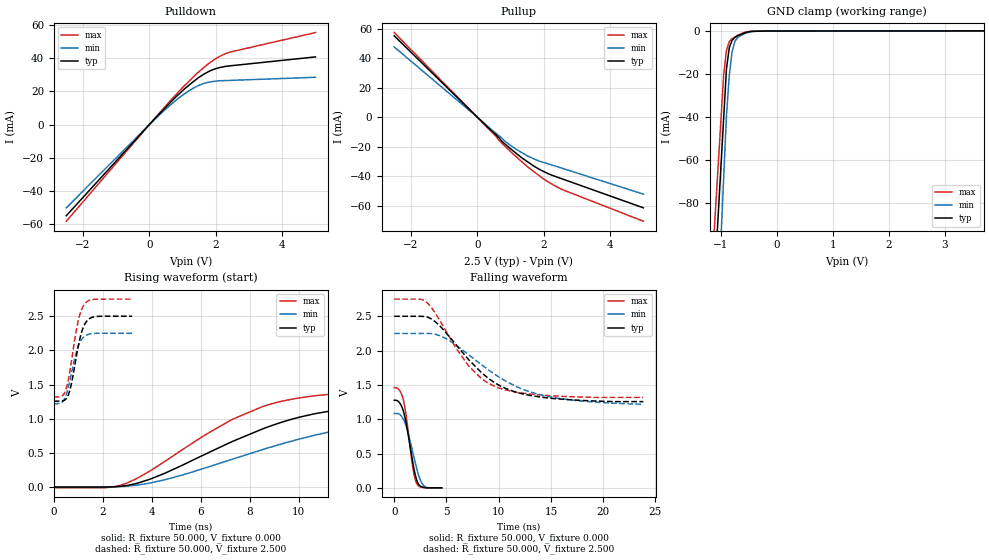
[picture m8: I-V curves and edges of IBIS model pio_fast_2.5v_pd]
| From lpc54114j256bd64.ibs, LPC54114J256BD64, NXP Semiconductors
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[Model]   pio_fast_2.5v_pd
Model_type I/O
Vinl=4.000E-01
Vinh=1.500E+00
Vref=0.000E+00
Rref=1.000E+06
Cref=2.000E-11
Vmeas=1.250E+00
C_comp   9.060E-12   8.700E-12   9.420E-12
[Voltage Range]   2.500E+00   2.250E+00   2.750E+00
[POWER Clamp Reference]   2.500E+00   2.250E+00   2.750E+00
[GND Clamp Reference]   0.000E+00   0.000E+00   0.000E+00
[Pullup Reference]   2.500E+00   2.250E+00   2.750E+00
[Pulldown Reference]   0.000E+00   0.000E+00   0.000E+00
[Temperature Range]   25   105   -40
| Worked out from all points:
|   slope of the pulldown table from 0 to 0.375 V, typ, clamps not added: 46.9 ohm
|   slope of the pullup table from 0 to 0.375 V, typ, clamps not added: 46.2 ohm
|   GND clamp passes 1 mA (typ) near -0.58 V on its own axis
|   rising waveform, R_fixture 50.000, V_fixture 0.000: 20-80 % time 5.17ns typ, 6.52ns min, 4.28ns max; typ from 0 V to 1.28 V
|   falling waveform, R_fixture 50.000, V_fixture 0.000: 20-80 % time 884ps typ, 1.06ns min, 766ps max; typ from 1.28 V to 0 V
|   rising waveform, R_fixture 50.000, V_fixture 2.500: 20-80 % time 409ps typ, 413ps min, 406ps max; typ from 1.26 V to 2.5 V
|   falling waveform, R_fixture 50.000, V_fixture 2.500: 20-80 % time 4.91ns typ, 6.27ns min, 4.01ns max; typ from 2.5 V to 1.26 V
[GND Clamp]
-2.5V     -757.5mA   -973.5mA   -687.5mA
-950mV    -40.89mA   -68.88mA   -20.67mA
-900mV    -17.78mA   -39.7mA    -9.038mA
-850mV    -7.888mA   -20.93mA   -4.915mA
-800mV    -4.357mA   -9.856mA   -3.541mA
-750mV    -3.031mA   -4.855mA   -2.756mA
-700mV    -2.227mA   -2.959mA   -1.97mA
-600mV    -1.164mA   -1.43mA    -872.3uA
-500mV    -329.3uA   -546.9uA   -245.1uA
-200mV    -21.96uA   -28.58uA   -10.55uA
5V        98.58uA    104.9uA    95.1uA
[Power Clamp]
-2.5V     0A         0A         0A
0V        0A         0A         0A
2.5V      0A         0A         0A
5V        0A         0A         0A
[Pullup]
-2.5V     55.17mA    47.6mA     57.37mA
0V        0A         0A         0A
820mV     -17.99mA   -16.12mA   -19.39mA
1.4V      -28.61mA   -24.91mA   -31.48mA
1.94V     -36.26mA   -30.42mA   -40.98mA
2.26V     -39.55mA   -32.62mA   -45.65mA
2.54V     -41.8mA    -34.63mA   -48.95mA
5V        -61.57mA   -52.31mA   -70.72mA
[Pulldown]
-2.5V     -54.85mA   -50.1mA    -58.2mA
0V        0A         0A         0A
500mV     10.6mA     9.452mA    11.41mA
1.04V     21.22mA    18.33mA    23.13mA
1.42V     27.38mA    22.99mA    30.62mA
1.64V     30.38mA    24.79mA    34.37mA
1.84V     32.48mA    25.72mA    37.54mA
2.12V     34.38mA    26.41mA    41.13mA
2.44V     35.42mA    26.64mA    43.72mA
5V        40.78mA    28.5mA     55.43mA
[Rising Waveform]
R_fixture = 50.000
V_fixture = 0.000
V_fixture_min = 0.000
V_fixture_max = 0.000
|  time   V(typ)   V(min)   V(max)
0s        414.1uV    590.5uV    -10.9mV
2.1ns     386.6uV    1.722mV    -9.946mV
2.9ns     18.65mV    11.76mV    47.42mV
4.5ns     197.1mV    104.1mV    367mV
7.35ns    675.7mV    414.4mV    999.4mV
8.6ns     860.5mV    556.1mV    1.186V
9.85ns    1.006V     685.1mV    1.294V
11.6ns    1.129V     831.5mV    1.368V
14.65ns   1.22V      976.4mV    1.423V
23.65ns   1.277V     1.084V     1.452V
[Falling Waveform]
R_fixture = 50.000
V_fixture = 0.000
V_fixture_min = 0.000
V_fixture_max = 0.000
|  time   V(typ)   V(min)   V(max)
0s        1.277V     1.084V     1.461V
500ps     1.243V     1.073V     1.423V
900ps     1.106V     994.3mV    1.264V
1.2ns     896.8mV    873.5mV    990.9mV
1.8ns     352mV      502.7mV    281.1mV
1.95ns    235.1mV    405.2mV    158.7mV
2.15ns    117.7mV    282.7mV    64.49mV
2.55ns    20.25mV    97.9mV     13.51mV
2.9ns     4.226mV    22.79mV    3.144mV
4.55ns    414.1uV    590.5uV    149.8uV
[Rising Waveform]
R_fixture = 50.000
V_fixture = 2.500
V_fixture_min = 2.250
V_fixture_max = 2.750
|  time   V(typ)   V(min)   V(max)
0s        1.257V     1.22V      1.318V
400ps     1.265V     1.268V     1.355V
500ps     1.289V     1.344V     1.432V
600ps     1.355V     1.47V      1.581V
750ps     1.566V     1.718V     1.912V
950ps     1.972V     2.011V     2.354V
1.1ns     2.223V     2.14V      2.565V
1.25ns    2.374V     2.205V     2.675V
1.65ns    2.492V     2.248V     2.747V
3.2ns     2.5V       2.25V      2.75V
[Falling Waveform]
R_fixture = 50.000
V_fixture = 2.500
V_fixture_min = 2.250
V_fixture_max = 2.750
|  time   V(typ)   V(min)   V(max)
0s        2.5V       2.25V      2.75V
2.5ns     2.5V       2.25V      2.749V
3.1ns     2.491V     2.251V     2.705V
4.7ns     2.305V     2.195V     2.352V
7.1ns     1.873V     1.942V     1.783V
8.35ns    1.68V      1.795V     1.593V
9.7ns     1.524V     1.648V     1.475V
12.25ns   1.371V     1.44V      1.381V
14.9ns    1.307V     1.327V     1.343V
23.85ns   1.257V     1.22V      1.318V
[Ramp]
dV/dt_r   7.6469E-01/5.1563E-09   6.4858E-01/6.5173E-09   8.7806E-01/4.2483E-09
dV/dt_f   7.4600E-01/4.9050E-09   6.1833E-01/6.2646E-09   8.5930E-01/3.9848E-09
R_load = 50
